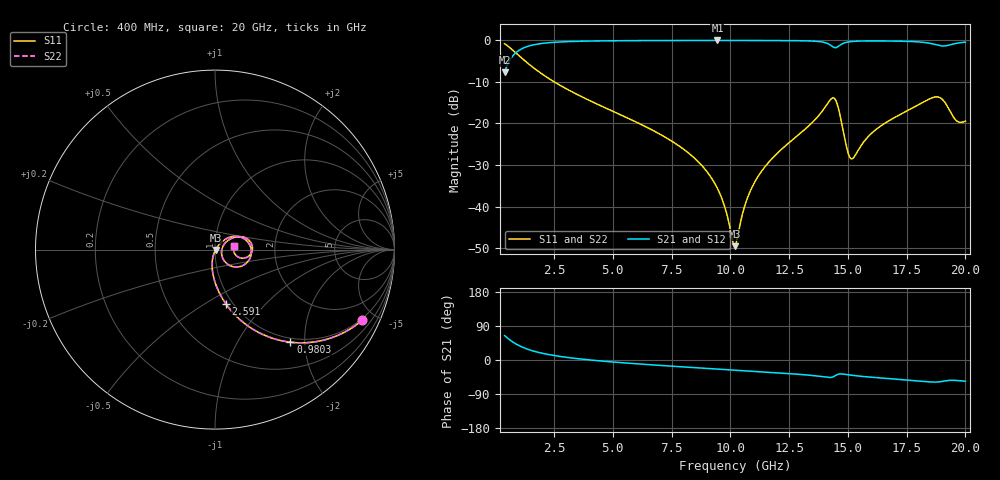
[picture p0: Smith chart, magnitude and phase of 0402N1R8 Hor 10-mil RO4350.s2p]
# GHz S MA R 50
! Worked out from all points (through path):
!   1960 points, 400 MHz to 20 GHz, reference 50 ohm
!   highest |S21| = -0.03 dB at 9.455 GHz (marker M1); lowest = -7.7 dB at 400 MHz (marker M2)
!   group delay of S21, straight-line fit = 12.4 ps
!   lowest |S11| = -49.5 dB at 10.18 GHz (marker M3), VSWR 1.01, Z = 50.3 - j0.159 ohm
!   |S11| at or under -10 dB: 2.514 GHz to end of sweep
!   |S22| runs from -49.5 to -0.8 dB; largest |S21 - S12| = 0
!   S11 on the Smith chart (normalised r, x): 400 MHz: 0.92, -4.22; 980.3 MHz: 0.93, -1.71; 2.591 GHz: 0.93, -0.62; 20 GHz: 1.23, +0.04
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0.4  0.91 -25.5  0.4142 64.4  0.4142 64.4  0.91 -25.5
0.9802961  0.665 -50.9  0.7461 39.1  0.7461 39.1  0.665 -50.9
1.640633  0.4649 -66.5  0.8842 23.3  0.8842 23.3  0.4649 -66.5
2.591118  0.3068 -78.8  0.9503 11.0  0.9503 11.0  0.3068 -78.8
3.671669  0.2103 -87.2  0.9758 2.4  0.9758 2.4  0.2103 -87.2
6.943338  0.07609 -102.2  0.9944 -14.0  0.9944 -14.0  0.07609 -102.2
8.51414  0.03742 -106.0  0.9961 -20.3  0.9961 -20.3  0.03742 -106.0
9.45462  0.01653 -103.2  0.9964 -23.9  0.9964 -23.9  0.01653 -103.2
10.18499  0.003346 -28.2  0.9962 -26.7  0.9962 -26.7  0.003346 -28.2
10.205  0.003373 -20.6  0.9962 -26.8  0.9962 -26.8  0.003373 -20.6
10.67524  0.01151 43.3  0.9959 -28.6  0.9959 -28.6  0.01151 43.3
11.1855  0.02317 49.8  0.9954 -30.6  0.9954 -30.6  0.02317 49.8
13.46667  0.1013 41.3  0.9804 -40.7  0.9804 -40.7  0.1013 41.3
14.09699  0.1672 22.9  0.9257 -45.4  0.9257 -45.4  0.1672 22.9
14.42716  0.2005 -14.3  0.8186 -42.8  0.8186 -42.8  0.2005 -14.3
14.60725  0.1488 -40.6  0.8508 -37.2  0.8508 -37.2  0.1488 -40.6
14.99745  0.04561 -35.5  0.9539 -38.8  0.9539 -38.8  0.04561 -35.5
15.16753  0.03754 -7.0  0.9678 -40.3  0.9678 -40.3  0.03754 -7.0
16.73834  0.1074 34.4  0.9814 -49.0  0.9814 -49.0  0.1074 34.4
18.76937  0.2089 3.3  0.8828 -58.2  0.8828 -58.2  0.2089 3.3
19.61981  0.1081 -8.8  0.9201 -54.0  0.9201 -54.0  0.1081 -8.8
20  0.1068 9.5  0.9503 -56.1  0.9503 -56.1  0.1068 9.5
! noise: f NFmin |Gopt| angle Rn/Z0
0.4  0.001278  0.8005  4.411  0.001326
2.571  0.005074  0.6799  8.256  0.00305
4.752  0.00808  0.6385  13.52  0.004162
6.933  0.01083  0.6151  18.87  0.0051
9.104  0.01362  0.6046  24.13  0.0061
11.29  0.01737  0.6178  29.33  0.007953
13.47  0.03495  0.7576  34.72  0.02662
15.64  0.04083  0.7625  40.12  0.03085
17.82  0.05071  0.7838  45.14  0.04118
20  0.07418  0.833  50.36  0.0769
